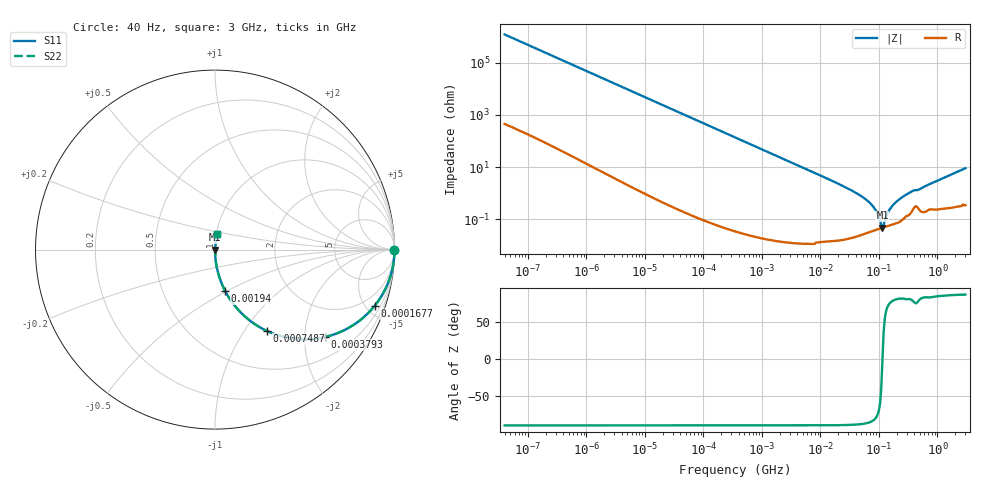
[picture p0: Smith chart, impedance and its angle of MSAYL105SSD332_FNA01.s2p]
! MSAYL105SSD332_FNA01  S-PARAMETER MODEL  ( General Type )
! Model Generated by TAIYO YUDEN Corporation (http://www.ty-top.com)
! Version 2.0
! TAIYO YUDEN Control No. 040624
! Copyright(c) 2004 TAIYO YUDEN CO.,LTD. All Rights Reserved.
! Product Description (link to TY-COMPAS)
! https://ds.yuden.co.jp/TYCOMPAS/or/detail?pn=MSAYL105SSD332KFNA01&u=M
! Products Name : Multilayer Ceramic Capacitors
! Characteristics :
!  Capacitance : 3300 pF , Rated Voltage : 10V
!  Case Size : 1.0 x 0.5 / 0.039 x 0.02 [mm/inch] , Thickness : 0.5 / 0.02 [mm/inch]
!  (Conditions: Temperature = 25 degC , DC Bias Current/Voltage = 0A / 0V)
! External Node Assignments :
!  1  o---| |---o  2
! GND o---------o GND
! Frequency Range : 40Hz  -  3GHz  [ 401 STEP ]
# MHz S RI R 50
! Freq[MHz].  S11 Real  S11 Imag  S21 Real  S21 Imag  S12 Real  S12 Imag  S22 Real  S22 Imag
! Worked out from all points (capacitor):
!   401 points, 40 Hz to 3 GHz, reference 50 ohm
!   read as one part in series: C = 3.33 nF near 44 Hz
!   lowest |Z| = 47.6 mohm at 114.7 MHz (marker M1)
!   series resonance near 114.9 MHz, so ESL is about 580 pH
!   S11 on the Smith chart (normalised r, x): 40 Hz: open; 167.7 kHz: 1.00, -5.69; 379.3 kHz: 1.00, -2.52; 748.7 kHz: 1.00, -1.28; 1.94 MHz: 1.00, -0.49; 3 GHz: 1.01, +0.18
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4e-05  1 -8.38e-05  3.8e-08 8.38e-05  3.8e-08 8.38e-05  1 -8.38e-05
5.3e-05  1 -0.000111  5.4e-08 0.000111  5.4e-08 0.000111  1 -0.000111
0.000834  1 -0.00175  3.56e-06 0.00175  3.56e-06 0.00175  1 -0.00175
0.017386  0.9987 -0.0364  0.00133 0.0364  0.00133 0.0364  0.9987 -0.0364
0.061867  0.9835 -0.1275  0.0165 0.1275  0.0165 0.1275  0.9835 -0.1275
0.167721  0.89 -0.3127  0.11 0.3127  0.11 0.3127  0.89 -0.3127
0.362475  0.6342 -0.4815  0.3658 0.4815  0.3658 0.4815  0.6342 -0.4815
0.379285  0.6129 -0.487  0.3871 0.487  0.3871 0.487  0.6129 -0.487
0.748653  0.289 -0.4532  0.711 0.4532  0.711 0.4532  0.289 -0.4532
1.939641  0.0572 -0.2319  0.9428 0.2319  0.9428 0.2319  0.0572 -0.2319
7.222098  0.00443 -0.0655  0.9956 0.0655  0.9956 0.0655  0.00443 -0.0655
28.13798  0.000424 -0.0159  0.9996 0.0159  0.9996 0.0159  0.000424 -0.0159
55.54024  0.000312 -0.00648  0.9997 0.00648  0.9997 0.00648  0.000312 -0.00648
83.52119  0.00038 -0.00262  0.9996 0.00262  0.9996 0.00262  0.00038 -0.00262
95.68847  0.000418 -0.00148  0.9996 0.00148  0.9996 0.00148  0.000418 -0.00148
104.7695  0.000446 -0.000743  0.9996 0.000743  0.9996 0.000743  0.000446 -0.000743
114.7124  0.000476 -1.38e-05  0.9995 1.38e-05  0.9995 1.38e-05  0.000476 -1.38e-05
125.5988  0.000508 0.000717  0.9995 -0.000717  0.9995 -0.000717  0.000508 0.000717
150.5692  0.000581 0.00221  0.9994 -0.00221  0.9994 -0.00221  0.000581 0.00221
206.7996  0.000749 0.00501  0.9993 -0.00501  0.9993 -0.00501  0.000749 0.00501
356.2883  0.00194 0.0112  0.9981 -0.0112  0.9981 -0.0112  0.00194 0.0112
3000  0.0114 0.0888  0.9886 -0.0888  0.9886 -0.0888  0.0114 0.0888
